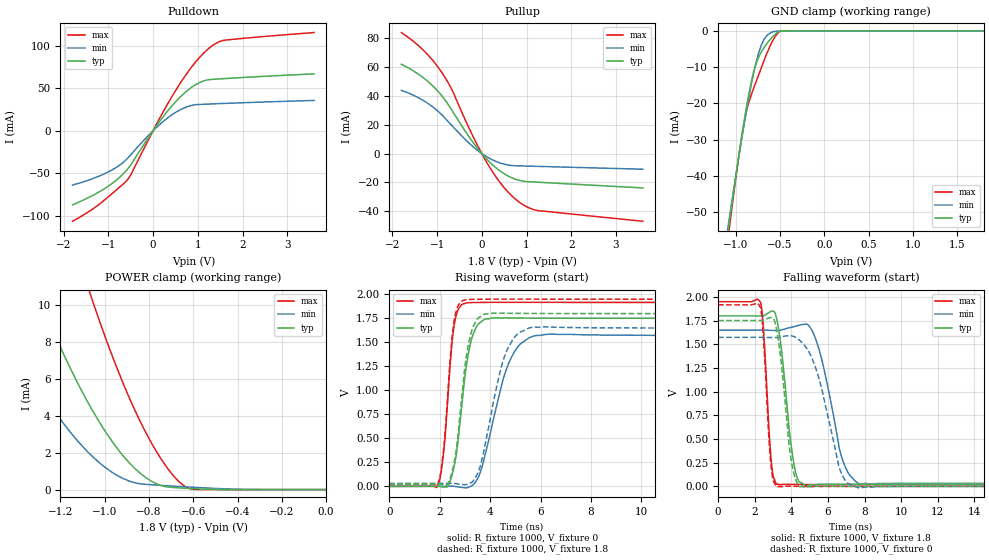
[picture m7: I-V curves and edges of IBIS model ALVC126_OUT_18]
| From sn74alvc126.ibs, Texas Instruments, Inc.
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[Model]   ALVC126_OUT_18
Model_type  3-state
Enable   Active-High
Vref =   0
Rref =   1000
Cref =   30p
Vmeas =   0.9
| variable   typ   min   max
C_comp   5.35pF   4.67pF   6.01pF
| C_pullup   6.33pF   5.11pF   6.91pF
| C_pulldown   9.77pF   5.21pF   16.21pF
| C_tri-state   5.35pF   4.67pF   6.01pF
[Temperature Range]   40   100   -40
| Ambient temperature   25   85   -40
[Voltage range]   1.8   1.65   1.95
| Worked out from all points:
|   slope of the pulldown table from 0 to 0.27 V, typ, clamps not added: 13.9 ohm
|   slope of the pullup table from 0 to 0.27 V, typ, clamps not added: 31.3 ohm
|   GND clamp passes 1 mA (typ) near -0.56 V on its own axis
|   POWER clamp passes 1 mA (typ) near -0.85 V on its own axis
|   rising waveform, R_fixture 1000, V_fixture 0: 20-80 % time 482ps typ, 914ps min, 337ps max; typ from 0 V to 1.75 V
|   falling waveform, R_fixture 1000, V_fixture 1.8: 20-80 % time 569ps typ, 1.01ns min, 337ps max; typ from 1.8 V to 0.023 V
|   rising waveform, R_fixture 1000, V_fixture 1.8: 20-80 % time 460ps typ, 798ps min, 332ps max; typ from 0.023 V to 1.8 V
|   falling waveform, R_fixture 1000, V_fixture 0: 20-80 % time 547ps typ, 1.17ns min, 330ps max; typ from 1.75 V to 0 V
[GND Clamp]
| ALVC126_OUT_18
|   Voltage   I(typ)   I(min)   I(max)
-1.8V     -193.2mA   -179.8mA   -208mA
-1.08V    -54.25mA   -52.87mA   -55.93mA
-1.065V   -51.58mA   -50.43mA   -53.01mA
-975mV    -36.05mA   -36.17mA   -36.32mA
-910mV    -25.63mA   -26.43mA   -26.02mA
-820mV    -13.54mA   -14.29mA   -17.31mA
-775mV    -9.388mA   -9.22mA    -14.32mA
-720mV    -6.206mA   -4.529mA   -10.76mA
-615mV    -2.473mA   -677.3uA   -4.329mA
-540mV    -660.7uA   -118.5uA   -1.081mA
-480mV    -21.04uA   -62.18uA   -16.51uA
1.8V      55.19pA    15.15nA    23.69pA
[POWER Clamp]
| ALVC126_OUT_18
|   Voltage   I(typ)   I(min)   I(max)
-1.8V     28.33mA    17.74mA    45.84mA
-1.53V    18.01mA    10.57mA    31.19mA
-1.3V     10.51mA    5.568mA    20.12mA
-1.18V    7.192mA    3.483mA    14.99mA
-1.06V    4.383mA    1.846mA    10.4mA
-990mV    3.016mA    1.131mA    8.007mA
-915mV    1.804mA    591.1uA    5.703mA
-835mV    838uA      308.1uA    3.577mA
-755mV    261uA      235.9uA    1.838mA
-685mV    110.2uA    183.9uA    684.3uA
-630mV    69.31uA    145.6uA    126uA
-16.28fV  55.19pA    338.7pA    25.85pA
[Pulldown]
| ALVC126_OUT_18
|   Voltage   I(typ)   I(min)   I(max)
-1.8V     -86.99mA   -63.73mA   -106.3mA
-1.375V   -76.65mA   -56.7mA    -92.8mA
-1.055V   -66.94mA   -49.73mA   -79.96mA
-775mV    -55.94mA   -41.39mA   -67.41mA
-570mV    -45.02mA   -32.35mA   -57.34mA
-485mV    -39.07mA   -27.35mA   -50.41mA
55mV      4.182mA    2.813mA    5.546mA
505mV     34.05mA    21.57mA    47.28mA
915mV     52.91mA    30.31mA    78.35mA
1.28V     60.17mA    31.45mA    98.11mA
1.605V    61.28mA    32.14mA    106.4mA
3.6V      66.82mA    35.6mA     115.3mA
[Pullup]
| ALVC126_OUT_18
|   Voltage   I(typ)   I(min)   I(max)
-1.8V     61.97mA    43.9mA     83.97mA
-1.315V   52.77mA    36.96mA    71.94mA
-1.105V   47.17mA    32.58mA    64.92mA
-915mV    40.83mA    27.53mA    57.19mA
-680mV    30.59mA    19.77mA    44.97mA
-240mV    9.612mA    5.999mA    14.7mA
125mV     -4.304mA   -2.484mA   -6.906mA
460mV     -13.17mA   -6.997mA   -22.15mA
800mV     -18.26mA   -8.462mA   -32.81mA
1.03V     -19.47mA   -8.666mA   -37.29mA
1.26V     -19.85mA   -8.867mA   -39.55mA
3.6V      -23.83mA   -10.83mA   -46.97mA
[Ramp]
| ALVC126_OUT_18
| variable   typ   min   max
dV/dt_r   1.06/4.94E-10   0.96/9.63E-10   1.16/3.41E-10
dV/dt_f   1.10/6.31E-10   1.01/1.11E-09   1.17/3.51E-10
R_load = 1000
[Rising Waveform]
| ALVC126_OUT_18
R_fixture =   1000
C_fixture =   0
L_fixture =   0
V_fixture =   0
V_fixture_min = 0
V_fixture_max = 0
|   Time   V(typ)   V(min)   V(max)
0s        25.37pV    2.694nV    19pV
1.935ns   1.267mV    198uV      12.8mV
2.17ns    -7.954mV   884.9uV    385.9mV
2.435ns   69.94mV    1.548mV    1.328V
2.58ns    215.8mV    -32.26uV   1.686V
3.1ns     1.325V     -13.08mV   1.913V
3.55ns    1.695V     103.2mV    1.916V
4.785ns   1.755V     1.31V      1.917V
5.82ns    1.752V     1.571V     1.917V
50ns      1.751V     1.573V     1.917V
[Falling Waveform]
| ALVC126_OUT_18
R_fixture =   1000
C_fixture =   0
L_fixture =   0
V_fixture =   1.8
V_fixture_min = 1.65
V_fixture_max = 1.95
|   Time   V(typ)   V(min)   V(max)
0s        1.8V       1.65V      1.95V
2.325ns   1.8V       1.65V      1.941V
2.915ns   1.849V     1.647V     245.4mV
3.235ns   1.741V     1.645V     20.16mV
4.15ns    230.9mV    1.686V     20.75mV
4.81ns    7.835mV    1.713V     19.04mV
5.59ns    22.8mV     1.395V     18.72mV
6.815ns   23.47mV    273.5mV    18.89mV
7.77ns    23.07mV    25.6mV     19mV
50ns      23.19mV    31.39mV    19.04mV
[Rising Waveform]
| ALVC126_OUT_18
R_fixture =   1000
C_fixture =   0
L_fixture =   0
V_fixture =   1.8
V_fixture_min = 1.65
V_fixture_max = 1.95
|   Time   V(typ)   V(min)   V(max)
0s        23.19mV    31.39mV    19.04mV
1.93ns    24.32mV    31.53mV    29.33mV
2.17ns    15.48mV    32.06mV    416.9mV
2.425ns   89.71mV    32.4mV     1.351V
2.575ns   247.1mV    30.75mV    1.727V
3.09ns    1.402V     19.92mV    1.947V
3.595ns   1.766V     197.1mV    1.949V
4.65ns    1.803V     1.405V     1.951V
5.68ns    1.801V     1.658V     1.95V
50ns      1.8V       1.65V      1.95V
[Falling Waveform]
| ALVC126_OUT_18
R_fixture =   1000
C_fixture =   0
L_fixture =   0
V_fixture =   0
V_fixture_min = 0
V_fixture_max = 0
|   Time   V(typ)   V(min)   V(max)
0s        1.751V     1.573V     1.917V
2.32ns    1.751V     1.574V     1.887V
2.87ns    1.783V     1.571V     264.9mV
3.23ns    1.624V     1.572V     -4.298mV
3.97ns    308.4mV    1.589V     1.972mV
4.49ns    -4.868mV   1.536V     463uV
5.405ns   443.5uV    1.21V      -293.8uV
6.695ns   21.23uV    158.4mV    -118.3uV
7.665ns   -132uV     -14.67mV   -34.44uV
50ns      10.33nV    12.67nV    -1.312nV
